VAR_GLOBAL
	
//	inputs 	AT%IB0 : ARRAY[0..20] OF BYTE;	// define used input space - not used 
//	outputs AT%QB0 : ARRAY[0..20] OF BYTE;	// define used output space - not used 
	memory 	AT%MB0 : ARRAY[0..20] OF BYTE;	// define used memory space
//	dddata	: ARRAY[0..20] OF BYTE;			// define used data space - not used 


//datapoints SLAVE -> MASTER (monitoring direction)
	(* Input IW0-9*)	// example

	(* Output QW0-9*)	// example
	
	(* Memory MW0-9*)	// example
		(*Single points*)
		bSlaveToMaster 	AT%MX0.0	: BOOL;	// obj addr: 10 - M_SP_NA_1 at byte/bit offset: 0/0
	
	(* Data *)	
		
//datapoints MASTER -> SLAVE (control directon)
	(* Input IW10-20*)	// example

	(* Output QW10-20*)	// example
	
	(* Memory MW10-20*)	// example
		(*Single points*)
		bMasterToSlave 	AT%MX5.0	: BOOL; // obj addr: 101 - C_SC_NA_1 at byte/bit offset: 5/0
		
	(* Data*)

//other variables
	
END_VAR
